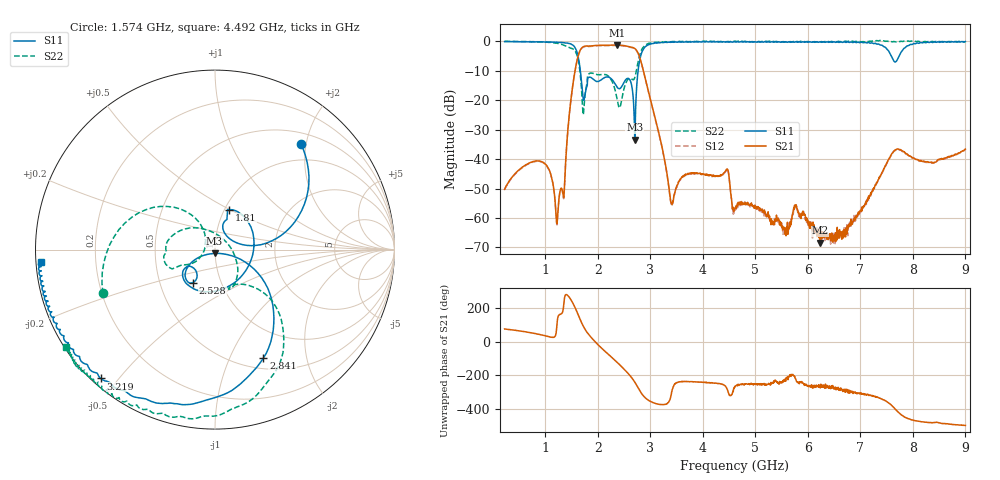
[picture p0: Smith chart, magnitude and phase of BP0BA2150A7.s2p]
!Agilent Technologies,E8358A,US41080443,A.07.50.56
!Agilent E8358A: A.07.50.56
!Date: Thursday, November 09, 2017 08:56:29
!Correction: S11(Full 2 Port(1,2))
!S21(Full 2 Port(1,2))
!S12(Full 2 Port(1,2))
!S22(Full 2 Port(1,2))
!S2P File: Measurements: S11, S21, S12, S22:
# Hz S  dB  R 50
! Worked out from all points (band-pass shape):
!   1601 points, 225 MHz to 9 GHz, reference 50 ohm
!   highest |S21| = -1.21 dB at 2.364 GHz (marker M1); lowest = -68.4 dB at 6.23 GHz (marker M2)
!   |S21| within 3 dB of the highest: 1.638 GHz to 2.773 GHz (1.135 GHz wide, 51.5 % of centre)
!   lowest |S11| = -33.4 dB at 2.704 GHz (marker M3), VSWR 1.04, Z = 49.7 - j2.12 ohm
!   |S11| at or under -10 dB: 1.667 GHz to 2.767 GHz (1.099 GHz wide, 49.6 % of centre)
!   |S22| runs from -24.9 to 0.3 dB; largest |S21 - S12| = 0.017
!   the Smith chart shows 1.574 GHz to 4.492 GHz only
!   S11 on the Smith chart (normalised r, x): 1.574 GHz: 0.69, +1.91; 1.81 GHz: 1.05, +0.50; 2.528 GHz: 0.73, -0.28; 2.841 GHz: 0.62, -1.34; 3.219 GHz: 0.02, -0.45; 4.492 GHz: 0.02, -0.04
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2.25e8  -0.09 172.3  -50.29 76.7  -50.36 76.2  0.01 168.3
9.27e8  -0.23 143.4  -40.87 41.4  -41.03 41.5  -0.22 120.2
1.234125e9  -0.32 121.0  -59.35 138.3  -59.65 141.5  -0.69 65.3
1.398656e9  -0.55 100.2  -37.61 -78.4  -37.75 -78.6  -1.64 -11.6
1.574156e9  -2.40 50.7  -9.18 -160.9  -9.29 -160.8  -3.47 -158.7
1.689328e9  -13.78 6.1  -2.32 114.6  -2.45 114.7  -16.12 119.8
1.809984e9  -12.50 70.4  -1.64 50.7  -1.79 51.0  -11.50 -156.8
2.023875e9  -13.52 -52.0  -1.35 -23.4  -1.48 -23.3  -11.34 -177.2
2.363906e9  -15.47 -146.4  -1.21 -120.5  -1.37 -120.3  -19.39 105.2
2.528438e9  -13.09 -123.9  -1.56 -171.7  -1.69 -171.6  -14.37 -49.4
2.703938e9  -33.40 -95.6  -2.43 120.2  -2.58 120.4  -12.29 -52.5
2.841047e9  -3.58 -66.0  -8.05 49.0  -8.20 49.2  -2.60 -61.7
3.153656e9  -0.44 -126.1  -30.53 -10.8  -30.67 -10.8  -0.25 -109.6
3.219469e9  -0.36 -131.6  -35.57 -13.6  -35.75 -13.3  -0.20 -114.2
3.411422e9  -0.23 -143.3  -55.00 63.5  -55.62 64.6  -0.06 -123.4
4.491844e9  -0.26 -175.9  -44.88 52.7  -45.08 51.5  -0.09 -146.7
4.6125e9  -0.20 -178.9  -56.62 90.5  -57.07 92.8  0.06 -148.4
6.076828e9  -0.28 144.6  -63.97 102.0  -64.76 85.5  -0.16 -176.1
6.230391e9  -0.13 140.4  -68.41 96.8  -64.45 95.9  -0.19 -178.9
7.541156e9  -3.36 48.3  -39.95 -4.4  -40.21 -4.0  -0.11 150.2
7.744078e9  -4.70 -114.6  -36.78 -64.9  -36.83 -64.9  -0.08 146.1
9e9  -0.05 147.0  -36.60 -137.6  -36.80 -137.2  -0.15 126.6
